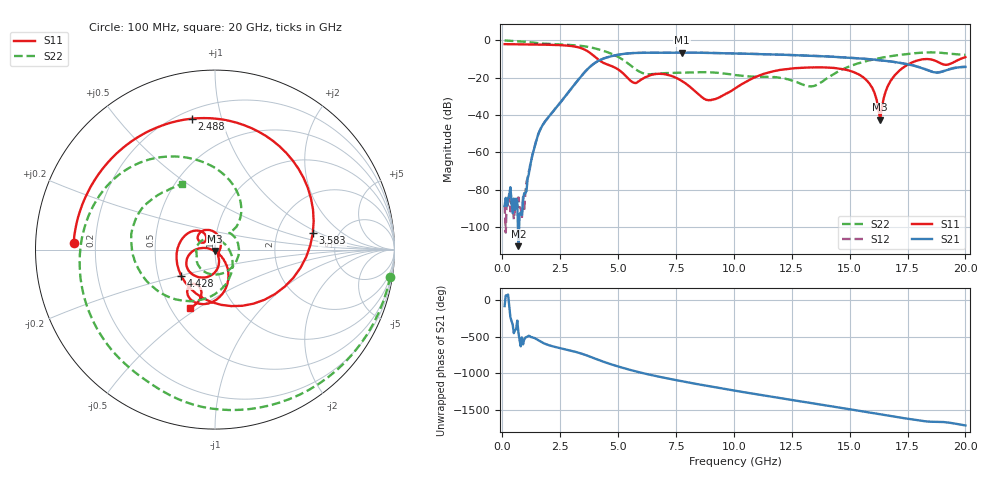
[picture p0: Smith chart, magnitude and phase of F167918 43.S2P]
!  2-Port S-parameters saved by WinCal
! VAR MeasName=S-Parameters (CALIBRATED_DATA) read from VNA (N5242A)
! VAR MeasDate=2016-11-22 10:26:52
! VAR NAME=F167918 43
! VAR FILENAME=F167918 43.S2P
! VAR DATE=2016-11-22 10:26:52
! VAR PHYS_PORTS=1,2
# Hz S DB R 50
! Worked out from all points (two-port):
!   401 points, 100 MHz to 20 GHz, reference 50 ohm
!   highest |S21| = -6.59 dB at 7.761 GHz (marker M1); lowest = -110.4 dB at 697 MHz (marker M2)
!   |S21| within 3 dB of the highest: 4.422 GHz to 15.29 GHz (10.87 GHz wide, 110 % of centre)
!   lowest |S11| = -42.5 dB at 16.32 GHz (marker M3), VSWR 1.02, Z = 49.7 - j0.701 ohm
!   |S11| at or under -10 dB: 4.112 GHz to 19.79 GHz (15.68 GHz wide, 131 % of centre)
!   |S22| runs from -24.7 to -0.1 dB; largest |S21 - S12| = 0.0051
!   S11 on the Smith chart (normalised r, x): 100 MHz: 0.12, +0.02; 2.488 GHz: 0.25, +0.81; 3.583 GHz: 3.22, +0.85; 4.428 GHz: 0.66, -0.21; 20 GHz: 0.62, -0.46
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1e8  -2.07 177.3  -88.86 -83.9  -88.33 171.0  -0.10 -8.8
6.97e8  -2.15 161.4  -110.38 -83.9  -84.22 124.2  -0.53 -56.2
1.04525e9  -2.21 151.8  -80.80 -146.1  -75.87 -135.6  -0.88 -81.2
1.64225e9  -2.32 133.7  -47.79 155.3  -47.74 154.5  -1.68 -117.9
2.488e9  -2.61 99.9  -33.69 65.2  -33.69 64.8  -2.22 -161.0
3.43325e9  -4.35 28.2  -18.88 -11.6  -18.90 -11.6  -3.04 152.4
3.5825e9  -5.15 9.5  -16.77 -27.6  -16.77 -27.4  -3.28 144.5
3.9805e9  -8.64 -54.6  -12.32 -74.7  -12.28 -74.6  -4.29 123.5
4.42825e9  -12.44 -141.8  -9.56 -127.0  -9.52 -127.2  -5.91 100.8
5.075e9  -16.27 136.6  -7.60 168.1  -7.61 167.8  -9.42 67.9
5.7715e9  -22.94 144.3  -6.75 107.4  -6.76 107.3  -15.73 47.0
6.7665e9  -17.96 130.3  -6.68 36.1  -6.69 35.9  -17.88 38.3
7.7615e9  -21.89 77.9  -6.59 -26.0  -6.62 -26.0  -17.40 -25.6
8.90575e9  -32.19 -20.2  -6.74 -92.5  -6.75 -92.5  -17.12 -104.0
1.005e10  -25.83 -66.8  -7.05 -154.7  -7.06 -154.5  -18.62 -150.5
1.1841e10  -16.26 -103.5  -7.69 112.7  -7.65 113.0  -19.80 168.7
1.338325e10  -14.59 -134.1  -8.34 35.1  -8.28 35.0  -24.63 52.8
1.547275e10  -18.84 -179.0  -9.78 -70.9  -9.80 -71.4  -11.97 -91.6
1.63185e10  -42.51 -109.9  -10.70 -114.9  -10.73 -114.3  -9.50 -121.6
1.67165e10  -22.94 -48.2  -11.24 -135.2  -11.31 -134.8  -8.64 -134.7
1.786075e10  -11.08 -88.5  -13.92 166.6  -13.82 167.0  -6.88 -172.7
2e10  -9.03 -113.2  -14.31 92.9  -14.15 92.6  -7.79 116.9
